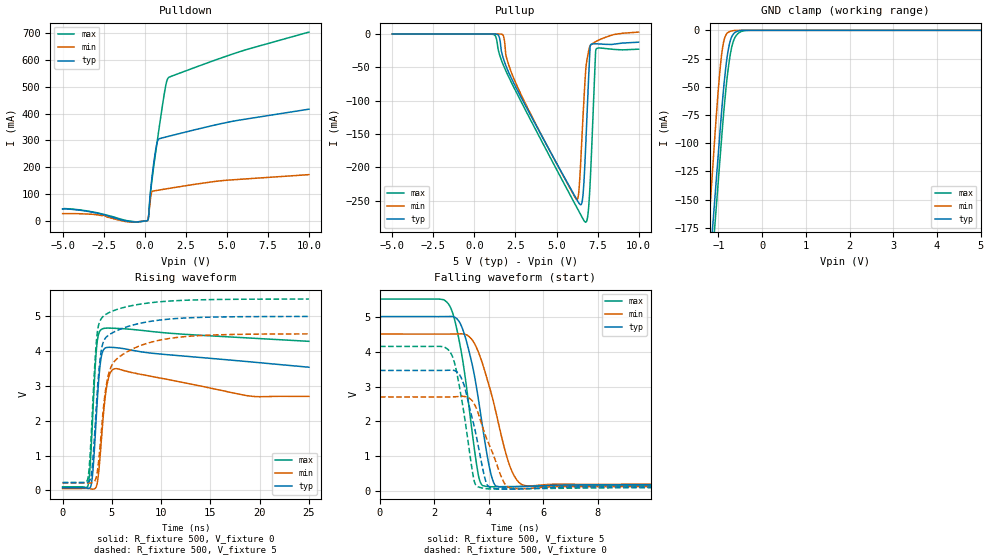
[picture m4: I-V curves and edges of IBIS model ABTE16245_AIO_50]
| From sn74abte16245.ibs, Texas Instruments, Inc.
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[Model]   ABTE16245_AIO_50
Model_type  I/O
Vinl=1.4
Vinh=1.6
Enable   Active-Low
Vref =   0
Rref =   500
Cref =   50p
Vmeas =   1.5
| variable   typ   min   max
C_comp   6.80pF   5.58pF   9.24pF
| C_pullup   7.28pF   5.89pF   10.00pF
| C_pulldown   5.43pF   1.13pF   11.65pF
| C_tri-state   6.80pF   5.58pF   9.24pF
[Temperature Range]   40   -40   100
| Ambient temperature   25   -40   85
[Voltage range]   5   4.5   5.5
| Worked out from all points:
|   slope of the pulldown table from 0 to 0.75 V, typ, clamps not added: 2.58 ohm
|   GND clamp passes 1 mA (typ) near -0.58 V on its own axis
|   rising waveform, R_fixture 500, V_fixture 0: 20-80 % time 448ps typ, 456ps min, 443ps max; typ from 0.078 V to 3.54 V
|   falling waveform, R_fixture 500, V_fixture 5: 20-80 % time 645ps typ, 860ps min, 582ps max; typ from 5 V to 0.216 V
|   rising waveform, R_fixture 500, V_fixture 5: 20-80 % time 792ps typ, 1.35ns min, 641ps max; typ from 0.224 V to 5 V
|   falling waveform, R_fixture 500, V_fixture 0: 20-80 % time 570ps typ, 731ps min, 494ps max; typ from 3.46 V to 0.091 V
[GND Clamp]
| ABTE16245_AIO_50
|   Voltage   I(typ)   I(min)   I(max)
-5V       -2.612A    -2.791A    -2.656A
-1.23V    -223.8mA   -178.5mA   -249.4mA
-1.18V    -198.5mA   -149.9mA   -223.2mA
-1.075V   -145.6mA   -90.12mA   -169.6mA
-1V       -107.9mA   -51.05mA   -131.9mA
-925mV    -70.79mA   -20.88mA   -94.45mA
-875mV    -48.82mA   -9.047mA   -71.16mA
-825mV    -30.65mA   -3.783mA   -50.65mA
-750mV    -12.42mA   -1.219mA   -26.56mA
-625mV    -2.021mA   -92.53uA   -6.512mA
-400mV    -6.82uA    -3.05nA    -168.6uA
5V        102.6pA    98.01pA    2.523nA
[Pulldown]
| ABTE16245_AIO_50
|   Voltage   I(typ)   I(min)   I(max)
-5V       44.88mA    27.06mA    43.64mA
-2.5V     23.13mA    20.84mA    24.45mA
-965mV    -2.15mA    -3.913mA   -373.3uA
160mV     735.5uA    661.1uA    1.224mA
235mV     14.9mA     17.72mA    15.14mA
420mV     148.9mA    105.7mA    140.1mA
590mV     232.3mA    111.9mA    221.2mA
755mV     291.4mA    113.6mA    293.1mA
1.22V     311.5mA    118.4mA    483.3mA
1.43V     314.7mA    120.5mA    532.6mA
5.705V    374.9mA    154.4mA    628.9mA
10V       416.2mA    172.2mA    703.5mA
[Pullup]
| ABTE16245_AIO_50
|   Voltage   I(typ)   I(min)   I(max)
-5V       -10.39pA   -10.66pA   -12.09pA
1.155V    -6.531uA   -407.6pA   -435.9uA
1.72V     -33.04mA   -933.6uA   -43.89mA
2.585V    -82.66mA   -77.12mA   -88.79mA
6.24V     -248.3mA   -248.3mA   -260.2mA
6.38V     -254mA     -230.4mA   -266.6mA
6.57V     -250.1mA   -145mA     -275.4mA
6.775V    -169.6mA   -55.14mA   -282.2mA
6.92V     -85.95mA   -29.9mA    -269.5mA
7.05V     -18.43mA   -17.76mA   -222.5mA
7.4V      -14.64mA   -11.13mA   -23.52mA
10V       -12.19mA   2.976mA    -22.67mA
[Ramp]
| ABTE16245_AIO_50
| variable   typ   min   max
dV/dt_r   2.43/5.47E-10   2.08/6.53E-10   2.75/4.98E-10
dV/dt_f   2.93/6.57E-10   2.61/8.76E-10   3.22/5.91E-10
R_load = 500
[Rising Waveform]
| ABTE16245_AIO_50
R_fixture =   500
C_fixture =   0
L_fixture =   0
V_fixture =   0
V_fixture_min = 0
V_fixture_max = 0
|   Time   V(typ)   V(min)   V(max)
0s        78.24mV    54.95mV    103mV
2.59ns    55.91mV    55.3mV     150.9mV
2.785ns   78.75mV    50.1mV     664.2mV
3.005ns   364mV      36.72mV    1.823V
3.435ns   2.184V     114.8mV    4.059V
3.71ns    3.32V      660.7mV    4.538V
3.965ns   3.889V     1.558V     4.632V
4.53ns    4.108V     3.068V     4.663V
5.295ns   4.104V     3.495V     4.658V
24.99ns   3.539V     2.7V       4.283V
[Falling Waveform]
| ABTE16245_AIO_50
R_fixture =   500
C_fixture =   0
L_fixture =   0
V_fixture =   5
V_fixture_min = 4.5
V_fixture_max = 5.5
|   Time   V(typ)   V(min)   V(max)
0s        5V         4.5V       5.5V
2.565ns   5.003V     4.499V     5.298V
2.83ns    4.932V     4.503V     4.61V
3.145ns   4.379V     4.484V     3.178V
3.58ns    2.806V     4.048V     617.3mV
3.785ns   1.758V     3.604V     162.3mV
4.225ns   180.5mV    2.375V     134.4mV
4.785ns   129.1mV    693.5mV    138.9mV
5.305ns   143.7mV    168.8mV    143.2mV
24.99ns   215.9mV    209.3mV    218.5mV
[Rising Waveform]
| ABTE16245_AIO_50
R_fixture =   500
C_fixture =   0
L_fixture =   0
V_fixture =   5
V_fixture_min = 4.5
V_fixture_max = 5.5
|   Time   V(typ)   V(min)   V(max)
0s        223.8mV    215mV      224mV
2.555ns   231.3mV    214.8mV    332.8mV
2.74ns    272.9mV    214.3mV    812mV
2.975ns   585.5mV    219.8mV    1.988V
3.48ns    2.676V     452.1mV    4.425V
3.86ns    3.892V     1.455V     4.905V
4.27ns    4.344V     2.693V     5.034V
5.22ns    4.552V     3.695V     5.17V
8.565ns   4.841V     4.225V     5.38V
24.99ns   4.998V     4.498V     5.498V
[Falling Waveform]
| ABTE16245_AIO_50
R_fixture =   500
C_fixture =   0
L_fixture =   0
V_fixture =   0
V_fixture_min = 0
V_fixture_max = 0
|   Time   V(typ)   V(min)   V(max)
0s        3.459V     2.701V     4.147V
2.56ns    3.466V     2.702V     4V
2.78ns    3.442V     2.708V     3.541V
3.08ns    3.058V     2.717V     2.254V
3.465ns   1.843V     2.499V     286.8mV
3.755ns   719mV      1.875V     98.01mV
3.985ns   142.2mV    1.378V     74.44mV
4.56ns    65.66mV    246.8mV    69.48mV
4.91ns    67.96mV    86.3mV     72.53mV
24.99ns   91.42mV    93.87mV    103.6mV
